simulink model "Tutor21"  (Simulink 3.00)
settings: Solver=ode45  SolverMode=SingleTasking  StartTime=0.0  StopTime=10  RelTol=1e-3  AbsTol=1e-3
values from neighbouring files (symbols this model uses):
  Au = [a0 a1;a2]    [data_id1.m]    (also in data_id2.m = [a0;[a1 a2]])
  Ay = [A0 A1;A2]    [data_id1.m]    (also in data_id2.m = A0)
  Bu = [b0;b1]    [data_id1.m]    (also in data_id2.m)
  By = [B0;B1]    [data_id1.m]    (also in data_id2.m)
  Cu = [c0 c1]/den(1)    [data_id1.m]    (also in data_id2.m = [c0 c1])
  Cy = [C0;C1]/den(1)    [data_id1.m]    (also in data_id2.m = [C0;C1])
  Du = zeros(in*(cit+1),in)    [data_id1.m]    (also in data_id2.m = zeros(cit*in,in))
  Dy = -[zeros(out,out);By]/den(1)    [data_id1.m]    (also in data_id2.m = [D1;D2])
libraries: simulink3 x1

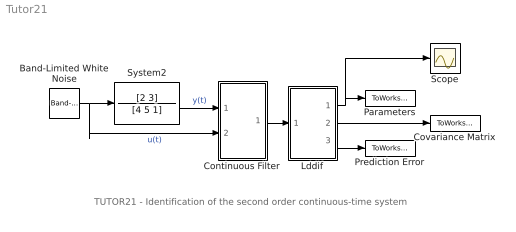
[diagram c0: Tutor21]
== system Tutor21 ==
  note: TUTOR21 - Identification of the second order continuous-time system
  Band-Limited White Noise : simulink3/Sources/Band-Limited White Noise  Cov=[0.1]  Ts=0.1  seed=[23341]
  Continuous Filter : Subsystem  mask(C-Filter){par=[1,1], cit=[1], men=[2], tc=[1]}
      mask prompts: par "No. of inputs and outputs -  [in,out]:"; cit "Numerator degree -  [dn]:"; men "Denominator degree -  [dd]:"; tc "Time constant of the filter - [Tc]:"
      mask help: C-filter: Continuous filters Authors: Lubos Cirka and Miroslav Fikar 1998 - 2004
      mask init:
      | in=par(1); out=par(2);  eval('data_id1');
  Covariance Matrix : ToWorkspace  VariableName=CovMatrix  SampleTime=0  SaveFormat=Matrix
  Lddif : Subsystem  mask(LDDIF){par=[4,1], L=[0.985], d=[0.01], poc=[0 0 0 0], kov=[10e6], ts=[1]}
      mask prompts: par "No. of estimated parameters and outputs - [n,m]:"; L "Exponential forgetting - [L]:"; d "Bittanti's correction - [d]:"; poc "Initial parameter estimates - [theta(1) ... theta(n)]:"; kov "Covariance matrix (see help, standard - [10e6]):"; ts "Sampling period - [ts]:"
      mask help: LDDIF: + Bittanti's corrections Authors: Lubos Cirka and Miroslav Fikar 1998 - 2004
      mask init:
      | n=par(1); m=par(2);
  Parameters : ToWorkspace  VariableName=BA  SampleTime=0  SaveFormat=Matrix
  Prediction Error : ToWorkspace  VariableName=PredError  SampleTime=0  SaveFormat=Matrix
  Scope : Scope
  System2 : TransferFcn  Numerator=[2 3]  Denominator=[4 5 1]
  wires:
  Lddif/2(covariance matrix) -> Covariance Matrix/1
  Lddif/3(prediction error) -> Prediction Error/1
  Lddif/1(theta) -> Parameters/1, Scope/1
  Band-Limited White Noise/1 -> Continuous Filter/2(u), System2/1  "u(t)"
  System2/1 -> Continuous Filter/1(y)  "y(t)"
  Continuous Filter/1("y, z") -> Lddif/1("y, z")

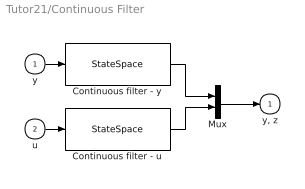
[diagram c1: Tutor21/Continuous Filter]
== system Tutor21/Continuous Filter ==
  y : Inport  Port=1  PortWidth=-1  SampleTime=-1  DataType=auto
  u : Inport  Port=2  PortWidth=-1  SampleTime=-1  DataType=auto
  Continuous filter - u : StateSpace  A=Au  B=Bu  C=Cu  D=Du  X0=0
  Continuous filter - y : StateSpace  A=Ay  B=By  C=Cy  D=Dy  X0=0
  Mux : Mux  Inputs=2
  "y, z" : Outport  Port=1  InitialOutput=0
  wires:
  y/1 -> Continuous filter - y/1
  u/1 -> Continuous filter - u/1
  Continuous filter - y/1 -> Mux/1
  Continuous filter - u/1 -> Mux/2
  Mux/1 -> "y, z"/1

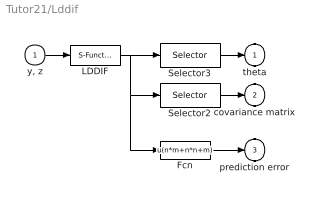
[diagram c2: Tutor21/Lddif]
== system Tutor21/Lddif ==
  "y, z" : Inport  Port=1  PortWidth=-1  SampleTime=-1  DataType=auto
  Fcn : Fcn  Expr=u(n*m+n*n+m)
  LDDIF : S-Function  FunctionName=lddif_s  Parameters=m, n, L, d, poc, kov, ts  PortCounts=[]  SFunctionModules=''
  Selector2 : Selector  Elements=[n*m:1:n*m+n*n]  InputPortWidth=n*m+n*n+m
  Selector3 : Selector  Elements=[1:1:n*m]  InputPortWidth=n*m+n*n+m
  theta : Outport  Port=1  InitialOutput=0
  covariance matrix : Outport  Port=2  InitialOutput=0
  prediction error : Outport  Port=3  InitialOutput=0
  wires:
  "y, z"/1 -> LDDIF/1
  LDDIF/1 -> Selector3/1, Selector2/1, Fcn/1
  Selector2/1 -> covariance matrix/1
  Selector3/1 -> theta/1
  Fcn/1 -> prediction error/1
